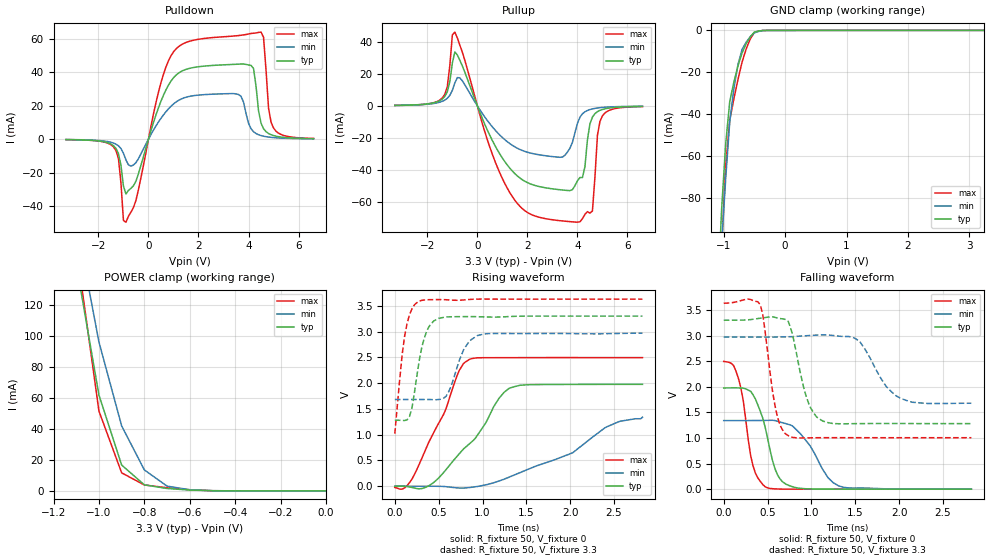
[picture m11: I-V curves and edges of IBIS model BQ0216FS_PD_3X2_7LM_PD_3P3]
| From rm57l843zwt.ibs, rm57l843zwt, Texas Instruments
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|   Model Cell FS_PD_3X2_7LM_PD_3P3
|BQ0216FS_PD_3X2_7LM_PD_3P3
[Model]   BQ0216FS_PD_3X2_7LM_PD_3P3
Model_type   I/O
Polarity   Non-Inverting
Enable   Active-Low
Vinl =  1.25
Vinh =  1.65
Cref =  15.0001pF
Rref =  101.0000M
Vref =  0V
Vmeas =  1.65
C_comp   1.2p   1.2p   1.2p
[Model Spec]
Vinl   1.25   1.12   1.38
Vinh   1.65   1.45   1.75
[Temperature Range]   25   155   -40
[Voltage Range]   3.3   2.97   3.63
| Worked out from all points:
|   slope of the pulldown table from 0 to 0.495 V, typ, clamps not added: 22 ohm
|   slope of the pullup table from 0 to 0.495 V, typ, clamps not added: 26.9 ohm
|   GND clamp passes 1 mA (typ) near -0.51 V on its own axis
|   POWER clamp passes 1 mA (typ) near -0.64 V on its own axis
|   rising waveform, R_fixture 50, V_fixture 0: 20-80 % time 523ps typ, 914ps min, 385ps max; typ from 0 V to 1.98 V
|   rising waveform, R_fixture 50, V_fixture 3.3: 20-80 % time 130ps typ, 167ps min, 107ps max; typ from 1.28 V to 3.3 V
|   falling waveform, R_fixture 50, V_fixture 0: 20-80 % time 182ps typ, 293ps min, 136ps max; typ from 1.98 V to 0 V
|   falling waveform, R_fixture 50, V_fixture 3.3: 20-80 % time 167ps typ, 275ps min, 128ps max; typ from 3.3 V to 1.28 V
[POWER_clamp]
|   voltage   I(typ)   I(min)   I(max)
-3.3V     2.372A     2.627A     3.149A
-1.1V     146.3mA    173.4mA    157.2mA
-1.067V   118.1mA    147.6mA    122mA
-1.033V   89.96mA    121.8mA    86.73mA
-1V       61.8mA     95.97mA    51.48mA
-900mV    16.69mA    41.94mA    11.68mA
-800mV    3.937mA    13.54mA    3.833mA
-700mV    1.574mA    3.091mA    2.066mA
-600mV    572.9uA    786.2uA    759.3uA
-500mV    114.1uA    194.7uA    140.7uA
0V        19.75uA    8.576uA    38.26uA
[Pulldown]
|   voltage   I(typ)   I(min)   I(max)
-3.3V     -267.3uA   -240.3uA   -277.5uA
-1.4V     -3.909mA   -2.325mA   -4.573mA
-1.2V     -8.625mA   -3.984mA   -11.65mA
-900mV    -32.84mA   -12.44mA   -49.75mA
1V        36.78mA    21.07mA    52.28mA
3.6V      44.94mA    26.74mA    62.08mA
4.1V      44.19mA    6.262mA    63.32mA
4.5V      9.589mA    2.146mA    64.15mA
4.6V      6.254mA    1.77mA     61.06mA
4.8V      3.393mA    1.259mA    18.58mA
5V        2.151mA    937.3uA    6.64mA
6.6V      305.4uA    234.7uA    420.4uA
[Pullup]
|   voltage   I(typ)   I(min)   I(max)
-3.3V     305.1uA    297.8uA    276.2uA
-1.4V     4.292mA    2.856mA    4.957mA
-900mV    33.76mA    14.39mA    46.19mA
500mV     -18.55mA   -11.22mA   -25.91mA
1.4V      -40.82mA   -24.72mA   -56.86mA
3.4V      -52.65mA   -32.06mA   -72.03mA
4V        -46.93mA   -10.94mA   -72.81mA
4.2V      -44.87mA   -4.98mA    -70.6mA
4.6V      -7.002mA   -1.879mA   -65.79mA
4.8V      -3.625mA   -1.322mA   -18.4mA
5V        -2.249mA   -979.1uA   -6.262mA
6.6V      -318.8uA   -256.1uA   -426.7uA
[GND_clamp]
|   voltage   I(typ)   I(min)   I(max)
-3.3V     -1.951A    -1.626A    -3.26A
-1.1V     -128.8mA   -138.1mA   -164.4mA
-1.033V   -85.86mA   -102.5mA   -105.1mA
-966.7mV  -54.21mA   -70.98mA   -64.57mA
-900mV    -33.86mA   -43.59mA   -42.8mA
-833.3mV  -24.67mA   -27.82mA   -32.66mA
-766.7mV  -16.98mA   -16.33mA   -23.45mA
-700mV    -10.78mA   -9.097mA   -15.17mA
-566.7mV  -3.082mA   -2.993mA   -4.123mA
-500mV    -821.5uA   -1.162mA   -950.4uA
-300mV    -7.829uA   -17.75uA   -10.85uA
3.233V    19.75uA    10.61uA    38.26uA
[Ramp]
| variable   typ   min   max
dV/dt_f   1.252892/0.1708794n  0.8050361/0.2801728n   1.628453/0.1291223n
dV/dt_r   1.216182/0.5377258n  0.8248212/0.9489635n   1.532758/0.3911993n
R_load = 50
[Rising Waveform]
R_fixture = 50
V_fixture = 0
V_fixture_min = 0
V_fixture_max = 0
|   time   V(typ)   V(min)   V(max)
0s        -84.57uV   184.2uV    -23.2mV
196ps     -24.53mV   367.4uV    139.4mV
444ps     73.74mV    -359uV     1.041V
584ps     321.8mV    -8.492mV   1.503V
736ps     631.3mV    -35.1mV    2.25V
852ps     824.5mV    -25.31mV   2.461V
1.308ns   1.904V     179.5mV    2.494V
2.028ns   1.975V     648.5mV    2.495V
2.412ns   1.976V     1.148V     2.495V
2.824ns   1.977V     1.339V     2.495V
[Rising Waveform]
R_fixture = 50
V_fixture = 3.3
V_fixture_min = 2.97
V_fixture_max = 3.63
|   time   V(typ)   V(min)   V(max)
0s        1.281V     1.682V     1.019V
112ps     1.275V     1.682V     2.912V
196ps     1.519V     1.682V     3.441V
280ps     2.45V      1.682V     3.591V
360ps     2.991V     1.682V     3.615V
444ps     3.205V     1.679V     3.62V
584ps     3.283V     1.743V     3.617V
784ps     3.29V      2.646V     3.613V
944ps     3.288V     2.923V     3.629V
2.824ns   3.3V       2.968V     3.63V
[Falling Waveform]
R_fixture = 50
V_fixture = 0
V_fixture_min = 0
V_fixture_max = 0
|   time   V(typ)   V(min)   V(max)
0s        1.976V     1.339V     2.494V
112ps     1.979V     1.339V     2.417V
168ps     1.977V     1.339V     2.164V
224ps     1.973V     1.339V     1.716V
332ps     1.848V     1.34V      471.5mV
472ps     1.216V     1.343V     48.9mV
612ps     284.9mV    1.326V     3.621mV
804ps     37.29mV    1.201V     406.3uV
1.308ns   923.6uV    66.14mV    63.89uV
2.824ns   82.84uV    622uV      -5.98uV
[Falling Waveform]
R_fixture = 50
V_fixture = 3.3
V_fixture_min = 2.97
V_fixture_max = 3.63
|   time   V(typ)   V(min)   V(max)
0s        3.3V       2.97V      3.63V
416ps     3.338V     2.97V      3.605V
612ps     3.343V     2.971V     1.418V
760ps     3.161V     2.977V     1.018V
944ps     1.797V     2.996V     1.001V
1.128ns   1.331V     3.014V     1.005V
1.548ns   1.28V      2.891V     1.005V
1.848ns   1.282V     2.016V     1.005V
2.028ns   1.281V     1.766V     1.005V
2.824ns   1.28V      1.678V     1.005V
